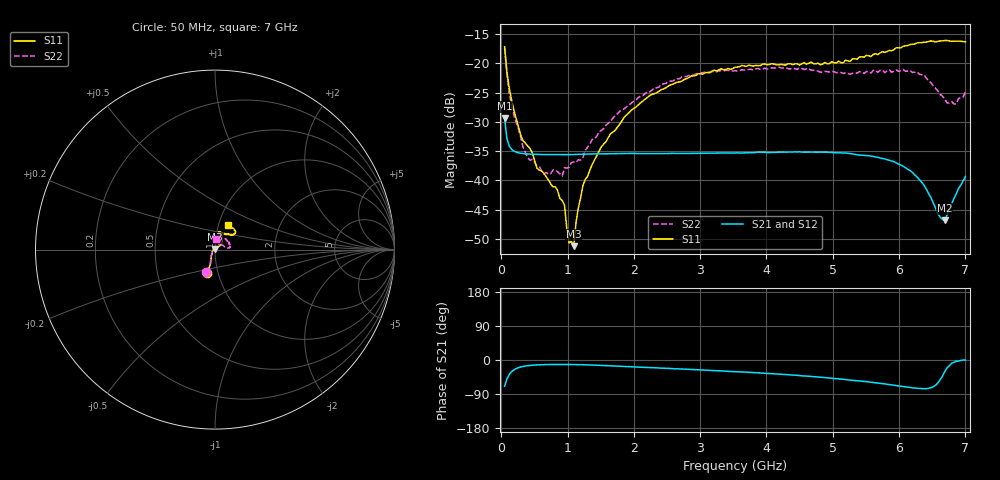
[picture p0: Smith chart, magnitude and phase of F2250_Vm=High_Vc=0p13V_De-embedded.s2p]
! Integrated Device Technology
! Corporate Headquarters
! 6024 Silver Creek Valley Road
! San Jose, CA 95138  USA
! Phone:  1-408-284-8200
! Toll Free:  1-800-223-1366
! Webpage:  http://www.idt.com/
! Timing and RF Division
! 515 Groton Road, Suite 102
! Westford, MA 01886-6024
! Device:  F2250
! Description: Voltage Variable RF Attenuator
! Frequency:  50.0 -  6000.00 MHz
! Package:  3x3 mm Thin QFN Plastic Package: 16 pin
! Ports:  2 RF, 3 DC
!  Pin  1  = GND
!  Pin  2  = NC
!  Pin  3  = RF1  = Port 1
!  Pin  4  = NC
!  Pin  5  = GND
!  Pin  6  = GND
!  Pin  7  = GND
!  Pin  8  = GND
!  Pin  9  = NC
!  Pin 10  = RF2  = Port 2
!  Pin 11  = NC
!  Pin 12  = GND
!  Pin 13  = GND
!  Pin 14  = VCNTRL
!  Pin 15  = VDD
!  Pin 16  = VMODE
! Vcntrl:  0.130 Volts
! Vmode:  +3.300 Volts
! Vdd:  +3.30  Volts
! Current:  1.245 mA
! Data:  The device was measured on a the F2250 evaluation board which has
!  individual transmission lines to the RF pins.  Data was collected
!  using a calibrated network analyzer.  The evaluation board was
!  de-embedded using a TRL calibration technique.
!  The reference plane is the edge of the package pin.
! Misc:  SN 10
!  Action Tracker AT0258
! Date Measured:  2014-11-26
! Date:  2015-10-15  MJV
! Note:
!  Integrated Device Technology supplies this data as a sample of measured
!  data at the package pin for this product.  Your particular data for this
!  product may vary.
!  Data was taken at 25 degrees C.
!  Integrated Device Technology reserves the right to change this data at anytime.
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# GHz S dB R 50
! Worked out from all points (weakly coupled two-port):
!   201 points, 50 MHz to 7 GHz, reference 50 ohm
!   highest |S21| = -29.38 dB at 50 MHz (marker M1); lowest = -46.8 dB at 6.687 GHz (marker M2)
!   lowest |S11| = -51.2 dB at 1.093 GHz (marker M3), VSWR 1.01, Z = 50 + j0.275 ohm
!   |S11| at or under -10 dB: start of sweep to end of sweep
!   |S22| runs from -39.2 to -17.4 dB; largest |S21 - S12| = 5e-05
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0.05  -17.18 -108.5  -29.38 -69.5  -29.38 -69.5  -17.37 -110.6
0.08475  -21.47 -107.4  -32.86 -50.1  -32.86 -50.1  -21.87 -109.0
0.15425  -26.23 -116.6  -34.68 -31.0  -34.68 -31.0  -27.10 -120.7
0.29325  -32.26 -127.4  -35.35 -18.4  -35.35 -18.4  -32.66 -133.5
0.3975  -34.11 -142.1  -35.47 -15.0  -35.48 -15.1  -36.08 -158.3
0.5365  -37.89 -154.7  -35.55 -12.9  -35.55 -12.9  -37.50 180.0
0.64075  -38.77 -162.4  -35.58 -12.2  -35.57 -12.2  -38.91 160.5
0.91875  -43.43 156.0  -35.60 -11.8  -35.60 -11.8  -39.25 127.8
0.9535  -44.22 170.9  -35.60 -11.8  -35.60 -11.8  -37.81 124.1
1.023  -50.66 141.1  -35.59 -11.9  -35.59 -11.9  -37.73 108.0
1.0925  -51.22 89.5  -35.57 -12.0  -35.57 -12.0  -36.84 98.9
1.12725  -47.18 62.0  -35.56 -12.1  -35.56 -12.1  -36.92 91.8
1.2315  -40.86 40.8  -35.52 -12.5  -35.52 -12.5  -36.07 77.2
1.6485  -32.02 41.2  -35.44 -15.1  -35.44 -15.2  -29.92 60.0
2.37825  -24.75 46.7  -35.40 -21.0  -35.40 -21.1  -24.03 53.9
3.525  -20.66 71.7  -35.32 -30.6  -35.32 -30.7  -21.26 72.9
4.7065  -20.06 72.0  -35.15 -43.9  -35.16 -43.9  -21.20 70.4
5.85325  -17.79 40.5  -36.58 -64.9  -36.58 -65.0  -21.13 23.4
6.27025  -16.53 39.4  -39.40 -74.5  -39.40 -74.6  -21.46 8.6
6.68725  -16.11 47.9  -46.80 -31.1  -46.79 -30.7  -26.03 28.5
6.861  -16.22 54.5  -42.30 -3.7  -42.27 -3.8  -26.96 57.4
7  -16.32 62.4  -39.35 -0.1  -39.32 -0.3  -24.81 83.7
